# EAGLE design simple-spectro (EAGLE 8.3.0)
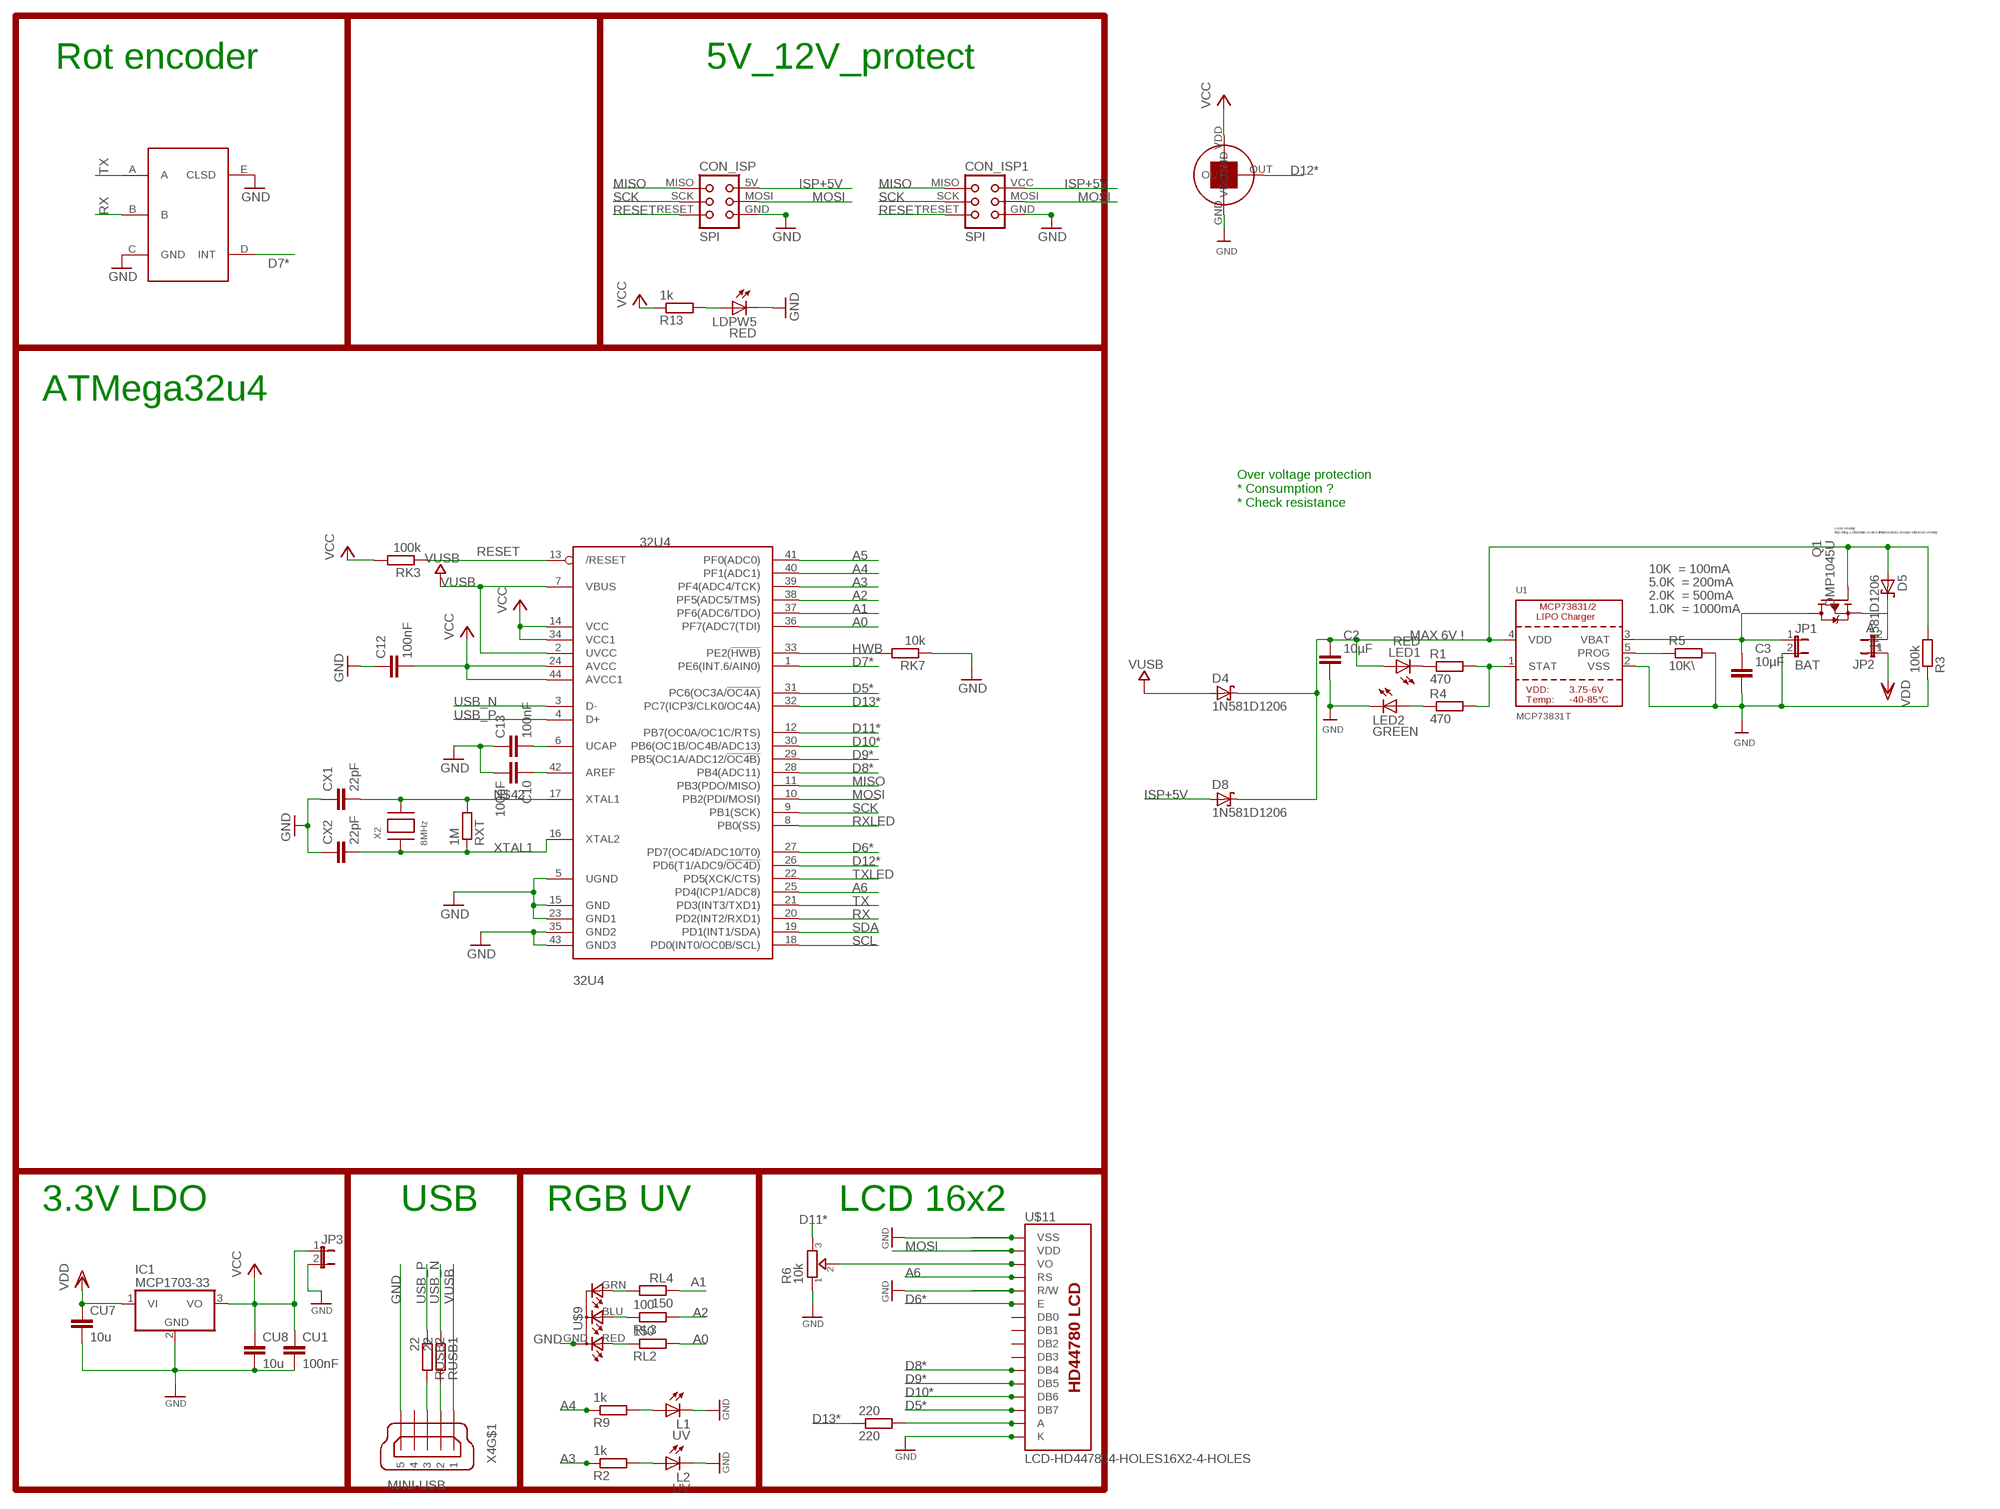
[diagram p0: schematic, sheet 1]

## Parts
32U4  32U4  ATMEGA32U4-AU  [TQFP44]
220  220  R-EU_M1206  [M1206]
C2  10µF  CAPACITOR_NPOL-1206  [C1206]
C3  10µF  CAPACITOR_NPOL-1206  [C1206]
C10  100nF  C-EUC1206  [C1206]
C12  100nF  C-EUC1206  [C1206]
C13  100nF  C-EUC1206  [C1206]
CON_ISP  SPI  TINYISPT  [TC2030-MCP-NL]
CON_ISP1  SPI  TINYISP  [TINYISP]
CU1  100nF  C-EUC1206  [C1206]
CU7  10u  C-EUC1206  [C1206]
CU8  10u  C-EUC1206  [C1206]
CX1  22pF  C-EUC1206  [C1206]
CX2  22pF  C-EUC1206  [C1206]
D4  1N581D1206  [LED-1206]
D5  1N581D1206  [LED-1206]
D8  1N581D1206  [LED-1206]
IC1  MCP1703-33  MCP1703DB  [SOT223]
JP1  BAT  JP1E  [JP1]
JP2  A  JP1E  [JP1]
JP3  JP1E  [JP1]
L1  UV  LED5MM  [LED5MM]
L2  UV  LED3MM  [LED3MM]
LDPW5  RED  LED1206  [LED-1206]
LED1  RED  LED1206  [LED-1206]
LED2  GREEN  LED1206  [LED-1206]
Q1  DMP1045U  TRANSISTOR_FET_TSM2301CX  [SOT-23]
R1  470  R-EU_M1206  [M1206]
R2  1k  R-EU_M1206  [M1206]
R3  100k  R-EU_M1206  [M1206]
R4  470  R-EU_M1206  [M1206]
R5  10K\  R-EU_M1206  [M1206]
R6  10k  TRIMMER-3362P  [TRIMMER_3362P]
R9  1k  R-EU_M1206  [M1206]
R13  1k  R-EU_M1206  [M1206]
RK3  100k  R-EU_M1206  [M1206]
RK7  10k  R-EU_M1206  [M1206]
RL2  150  R-EU_M1206  [M1206]
RL3  100  R-EU_M1206  [M1206]
RL4  150  R-EU_M1206  [M1206]
RUSB1  22  R-EU_M1206  [M1206]
RUSB2  22  R-EU_M1206  [M1206]
RXT  1M  R-EU_M1206  [M1206]
U1  MCP73831T  MCP73831/2  [SOT23-5]
U$1  EC11E  [EC11E]
U$7  TSL237  [TSL237]
U$9  RGB-COMMON-CATHODE  [LED-TRICOLOR-THROUGHHOLE]
U$11  LCD-HD447804-HOLES16X2-4-HOLES  [LCD-16X2-4HOLES]
X2  8MHz  XTALNX6035  [NX6035]
X4  MINI-USB  MINI-USB-SCHIELD-32005-201  [32005-201]

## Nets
A0: 32U4.36(PF7(ADC7(TDI)) RL2.2
A1: 32U4.37(PF6(ADC6/TDO)) RL4.1
A2: 32U4.38(PF5(ADC5/TMS)) RL3.2
A3: 32U4.39(PF4(ADC4/TCK)) R2.1
A4: 32U4.40(PF1(ADC1)) R9.1
A5: 32U4.41(PF0(ADC0))
A6: 32U4.25(PD4(ICP1/ADC8)) U$11.4(RS)
AREF: 32U4.42(AREF) C10.1
D5*: 32U4.31(PC6(OC3A/!OC4A)) U$11.14(DB7)
D6*: 32U4.27(PD7(OC4D/ADC10/T0)) U$11.6(E)
D7*: 32U4.1(PE6(INT.6/AIN0)) U$1.D(INT)
D8*: 32U4.28(PB4(ADC11)) U$11.11(DB4)
D9*: 32U4.29(PB5(OC1A/ADC12/!OC4B)) U$11.12(DB5)
D10*: 32U4.30(PB6(OC1B/OC4B/ADC13)) U$11.13(DB6)
D11*: 32U4.12(PB7(OC0A/OC1C/RTS)) R6.3
D12*: 32U4.26(PD6(T1/ADC9/!OC4D)) U$7.OUT
D13*: 32U4.32(PC7(ICP3/CLK0/OC4A)) 220.1
GND [power]: 32U4.5(UGND) 32U4.15(GND) 32U4.23(GND1) 32U4.35(GND2) 32U4.43(GND3) C2.2 C3.2 C10.2 C12.1 C13.1 CON_ISP1.GND CON_ISP.GND CU1.2 CU7.2 CU8.2 CX1.1 CX2.1 IC1.2(GND) JP1.2 JP3.2 L1.K(C) L2.K(C) LDPW5.C LED2.C R3.1 R5.2 R6.1 RK7.1 U1.2(VSS) U$1.C(GND) U$1.E(CLSD) U$7.GND U$9.GND(A2) U$11.1(VSS) U$11.5(R/W) U$11.16(K) X4.5
HWB: 32U4.33(PE2(!HWB)) RK7.2
ISP+5V: CON_ISP1.VCC CON_ISP.5V(VCC) D8.A
MISO: 32U4.11(PB3(PDO/MISO)) CON_ISP1.MISO CON_ISP.MISO
MOSI: 32U4.10(PB2(PDI/MOSI)) CON_ISP1.MOSI CON_ISP.MOSI U$11.2(VDD)
N$1: 32U4.6(UCAP) C13.2
N$2: R6.2 U$11.3(VO)
N$3: L1.A R9.2
N$4: LED1.C R1.1
N$5: R1.2 R4.2 U1.1(STAT)
N$6: R5.1 U1.5(PROG)
N$7: LED2.A R4.1
N$8: L2.A R2.2
N$9: RL4.2 U$9.GRN(CGREEN)
N$10: RL3.1 U$9.BLU(CBLUE)
N$11: 220.2 U$11.15(A)
N$12: LDPW5.A R13.2
N$13: RL2.1 U$9.RED(CRED)
N$15: C2.1 D4.C D5.A D8.C LED1.A Q1.1(G) R3.2 U1.4(VDD)
N$17 [power]: D5.C JP2.2 Q1.2(S)
N$42: 32U4.17(XTAL1) CX1.2 RXT.2 X2.P$2
RESET: 32U4.13(/RESET) CON_ISP1.RESET CON_ISP.RESET RK3.1
RX: 32U4.20(PD2(INT2/RXD1)) U$1.B
RXLED: 32U4.8(PB0(SS))
SCK: 32U4.9(PB1(SCK)) CON_ISP1.SCK CON_ISP.SCK
SCL: 32U4.18(PD0(INT0/OC0B/SCL))
SDA: 32U4.19(PD1(INT1/SDA))
TX: 32U4.21(PD3(INT3/TXD1)) U$1.A
TXLED: 32U4.22(PD5(XCK/CTS))
USB_N: 32U4.3(D-) RUSB1.1
USB_P: 32U4.4(D+) RUSB2.1
USBC_N: RUSB1.2 X4.2
USBC_P: RUSB2.2 X4.3
VBAT1: C3.1 JP1.1 Q1.3(D) U1.3(VBAT)
VCC: 32U4.14(VCC) 32U4.24(AVCC) 32U4.34(VCC1) 32U4.44(AVCC1) C12.2 CU1.1 CU8.1 IC1.3(VO) JP3.1 R13.1 RK3.2 U$7.VDD
VDD [power]: CU7.1 IC1.1(VI) JP2.1
VUSB: 32U4.2(UVCC) 32U4.7(VBUS) D4.A X4.1
XTAL1: 32U4.16(XTAL2) CX2.2 RXT.1 X2.P$1
Unconnected: U$11.7(DB0) U$11.8(DB1) U$11.9(DB2) U$11.10(DB3) X4.4 X4.M1(S:S1) X4.M2(S:S2) X4.M3(S:S3) X4.M4(S:S4)

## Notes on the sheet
- Rot encoder | 5V_12V_protect
- ATMega32u4
- Over voltage protection
  * Consumption ?
  * Check resistance
- Load sharing:
  http://blog.zakkemble.co.uk/a-lithium-battery-charger-with-load-sharing/
- 10K  = 100mA
- 5.0K  = 200mA
- 2.0K  = 500mA
- 1.0K  = 1000mA
- MAX 6V !
- 3.3V LDO | USB | RGB UV | LCD 16x2

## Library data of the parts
32U4 = adafruit:ATMEGA32U4: http://www.ladyada.net/library/eagle
220 R1-R5 R9 R13 RK3 RK7 RL2-RL4 RUSB1 RUSB2 RXT = rcl:R-EU_: RESISTOR, European symbol
C2 C3 = dp_devices:CAPACITOR_NPOL: Non-Polarized capacitor in various packages
C10 C12 C13 CU1 CU7 CU8 CX1 CX2 = resistor:C-EU: CAPACITOR, European symbol
CON_ISP = lpatiny:TINYISP: CONNECTOR
CON_ISP1 = lpatiny:TINYISP: CONNECTOR; OC_FARNELL: unknown; OC_NEWARK: unknown
D4 D5 D8 = lpatiny:1N581*: 1.0A SCHOTTKY BARRIER RECTIFIER
IC1 = linear:MCP1703: 250 mA, 16V, Low Quiescent Current LDO Regulator Source: http://ww1.microchip.com/downloads/en/DeviceDoc/22049b.pdf
JP1-JP3 = jumper:JP1E: JUMPER
L1 LDPW5 LED1 LED2 = SparkFun:LED: LEDs
L2 = led:LED: LED
Q1 = dp_devices:TRANSISTOR_FET_TSM2301CX: 20V P-Channel Enhancement Mode MOSFET
R6 = dp_devices:TRIMMER: Trimmer resistor
U1 = microbuilder:MCP73831/2: MCP73831/2 LIPO Charger VDD: 3.75 - 6V Temp -40 - 85°C Programmable Charge Rate: 15-500mA NOTE: STAT is a tri-state logic output on the MCP73831 and an open-drain output on the MCP73832. SOT23-5 with 4.2V output and tri-state logic on STAT = MCP73831T-2ACI/OT
U$1 = lpatiny:EC11E: ALPS Rotary encoder
U$7 = lpatiny:TSL237
U$9 = lpatiny:RGB-COMMON-CATHODE
U$11 = HD44780LCD:LCD-HD44780
X2 = lpatiny:XTAL: Low cost SMT crystals, no capacitors included
X4 = con-cypressindustries:MINI-USB-SCHIELD-: MINI USB-B Conector Source: www.cypressindustries.com; OC_FARNELL: unknown; OC_NEWARK: unknown

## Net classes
0 default: width 0.406 mm, clearance 0.25 mm
1 power: width 0.406 mm, drill 0.305 mm, clearance 0.25 mm
2 VIN: width 0.406 mm, clearance 0.25 mm
3 fine: width 0.406 mm, clearance 0.25 mm
4 aref: width 0.406 mm, clearance 0.25 mm

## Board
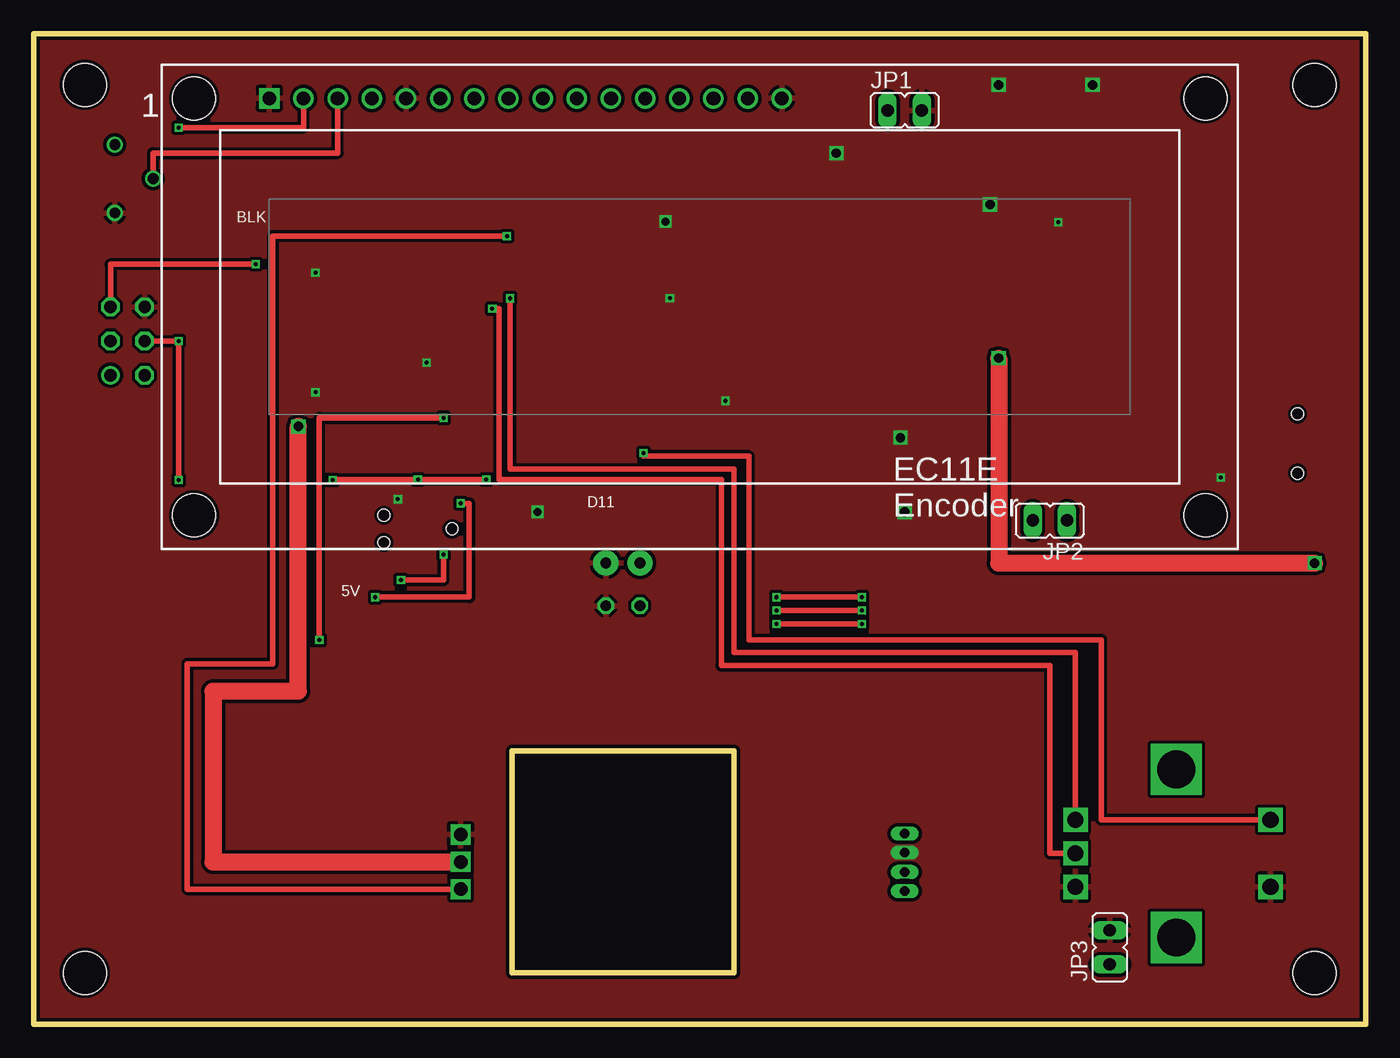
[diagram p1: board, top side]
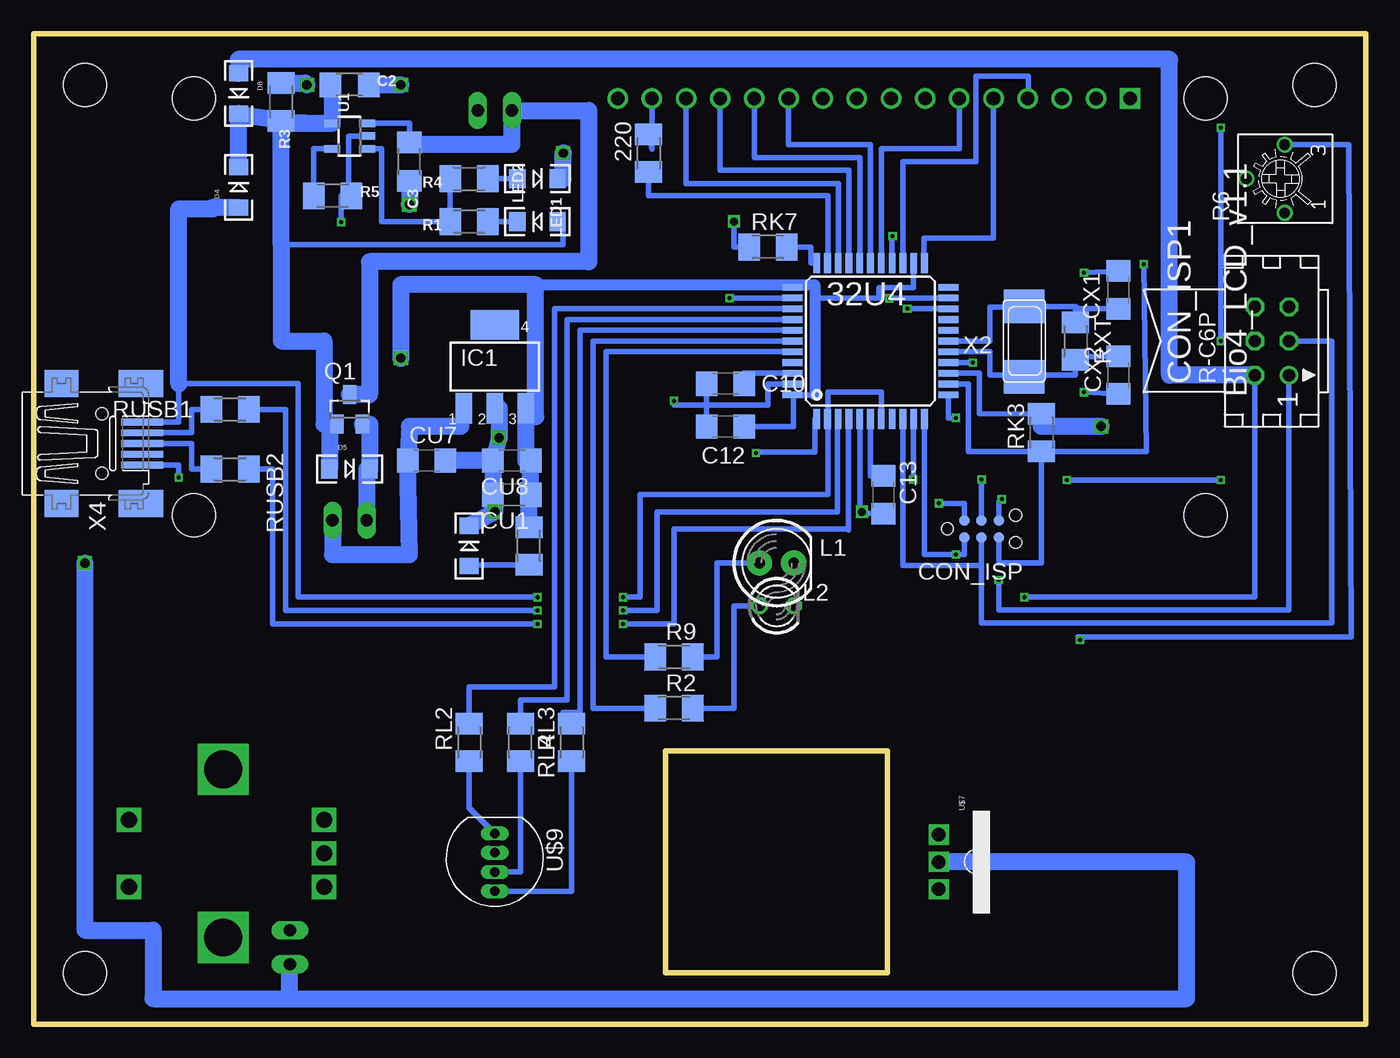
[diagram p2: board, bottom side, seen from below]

Size 99.06 x 73.66 mm. Coordinates in mm from the lower left corner, seen from the top.
Outline: 0,73.66 0,0 99.06,0 99.06,73.66 0,73.66
Outline: 35.56,20.32 52.07,20.32 52.07,3.81 35.56,3.81 35.56,20.32
Copper layers (1*2*15*16): Top 0.035mm / dielectric 0.2mm / layer 2 0.0175mm / dielectric 1.1mm / layer 15 0.0175mm / dielectric 0.2mm / Bottom 0.035mm
Design rules "SeeedStudio_DRU_no_angle_20130527": minimum track width 6mil, minimum drill 12mil, track to track 6mil, track to pad 6mil, pad to pad 6mil, via to via 6mil, smd to smd 0mil, copper to edge 10mil, drill to drill 10mil, minimum pad ring 6mil, minimum via ring 6mil, stop-mask expansion 2mil, vias tented up to drill 25mil, thermal gap 10mil
Holes 3.2 mm at 3.81,69.85 3.81,3.81 95.25,69.85 95.25,3.81

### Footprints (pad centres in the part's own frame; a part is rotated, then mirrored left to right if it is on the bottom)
TQFP44 = smd 1.5 x 0.5: 1 -5.8,4; 2 -5.8,3.2; 3 -5.8,2.4; 4 -5.8,1.6; 5 -5.8,0.8; 6 -5.8,0; 7 -5.8,-0.8; 8 -5.8,-1.6; 9 -5.8,-2.4; 10 -5.8,-3.2; 11 -5.8,-4; 23 5.8,-4; 24 5.8,-3.2; 25 5.8,-2.4; 26 5.8,-1.6; 27 5.8,-0.8; 28 5.8,0; 29 5.8,0.8; 30 5.8,1.6; 31 5.8,2.4; 32 5.8,3.2; 33 5.8,4 | smd 0.5 x 1.5: 12 -4,-5.8; 13 -3.2,-5.8; 14 -2.4,-5.8; 15 -1.6,-5.8; 16 -0.8,-5.8; 17 0,-5.8; 18 0.8,-5.8; 19 1.6,-5.8; 20 2.4,-5.8; 21 3.2,-5.8; 22 4,-5.8; 34 4,5.8; 35 3.2,5.8; 36 2.4,5.8; 37 1.6,5.8; 38 0.8,5.8; 39 0,5.8; 40 -0.8,5.8; 41 -1.6,5.8; 42 -2.4,5.8; 43 -3.2,5.8; 44 -4,5.8
M1206 = smd 1.6 x 2: 1 -1.4,0; 2 1.4,0
C1206 = smd 1.6 x 1.803: 1 -1.422,0; 2 1.422,0
C1206' = smd 1.6 x 1.8: 1 -1.4,0; 2 1.4,0
TC2030-MCP-NL = smd 0.787 x 0.787: 5V 1.27,0.635; GND 3.81,0.635; MISO 1.27,-0.635; MOSI 2.54,0.635; RESET 3.81,-0.635; SCK 2.54,-0.635 | hole 0.889: 0,0; 5.08,-1.016; 5.08,1.016
TINYISP = drill 0.914 octagon: GND 2.54,1.27; MOSI 0,1.27; RESET 2.54,-1.27; SCK 0,-1.27; VCC -2.54,1.27 | drill 0.914: MISO -2.54,-1.27
LED-1206 = smd 1.2 x 1.4: A -1.5,0; C 1.5,0
SOT223 = smd 1.219 x 2.235: 1 -2.311,-3.099; 2 0,-3.099; 3 2.311,-3.099 | smd 3.6 x 2.2: 4 0,3.099
JP1 = drill 0.914 long: 1 0,-1.27; 2 0,1.27
LED5MM = drill 0.813 pad 1.88: A -1.27,0; K 1.27,0
LED3MM = drill 0.813 octagon: A -1.27,0; K 1.27,0
SOT-23 = smd 1 x 1.4: 1 -0.95,-1.1; 2 0.95,-1.1; 3 0,1.1
TRIMMER_3362P = drill 0.8: 1 -2.54,-0.31; 2 0,2.54; 3 2.54,-0.31
SOT23-5 = smd 0.55 x 1.2: 1 -0.95,-1.3; 2 0,-1.3; 3 0.95,-1.3; 4 0.95,1.3; 5 -0.95,1.3
EC11E = drill 1.2 square: A -2.5,0; B 0,0; C 2.5,0; D -2.5,14.5; E 2.5,14.5 | drill 2.8 square: P$1 6.25,7.5; P$2 -6.25,7.5
TSL237 = drill 1 pad 1.27 square: GND -2.032,-2.54; OUT 2.032,-2.54; VDD 0,-2.54
LED-TRICOLOR-THROUGHHOLE = drill 0.7 long: BLU 2.175,0; GND -0.682,0; GRN 0.746,0; RED -2.111,0
LCD-16X2-4HOLES = drill 1.016 square: 1 -32,15.5 | drill 1.016: 2 -29.46,15.5; 3 -26.92,15.5; 4 -24.38,15.5; 5 -21.84,15.5; 6 -19.3,15.5; 7 -16.76,15.5; 8 -14.22,15.5; 9 -11.68,15.5; 10 -9.14,15.5; 11 -6.6,15.5; 12 -4.06,15.5; 13 -1.52,15.5; 14 1.02,15.5; 15 3.56,15.5; 16 6.1,15.5 | hole 3.2: -37.6,15.5; -37.6,-15.5; 37.6,-15.5; 37.6,15.5
NX6035 = smd 2.5 x 3: P$1 2.665,0; P$2 -2.565,0
32005-201 = smd 3.1 x 0.5: 1 3,1.6; 2 3,0.8; 3 3,0; 4 3,-0.8; 5 3,-1.6 | smd 2.5 x 2: M1 -3,-4.45; M2 -3,4.45 | smd 3.3 x 2: M3 2.9,4.45; M4 2.9,-4.45 | hole 0.9: 0,2.2; 0,-2.2

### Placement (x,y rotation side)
32U4  36.83,50.8 90 bottom
220  53.34,64.77 90 bottom
C2  75.56,69.85 0 bottom
C3  71.12,64.14 270 bottom
C10  100nF  [C1206']  47.62,47.62 180 bottom
C12  100nF  [C1206']  47.62,44.45 0 bottom
C13  100nF  [C1206']  35.88,39.37 90 bottom
CON_ISP  31.11,36.83 0 bottom
CON_ISP1  6.99,50.8 90 bottom
CU1  100nF  [C1206']  63.5,39.37 180 bottom
CU7  10u  [C1206']  69.85,41.91 0 bottom
CU8  10u  [C1206']  63.5,41.91 180 bottom
CX1  22pF  [C1206']  18.41,54.61 270 bottom
CX2  22pF  [C1206']  18.41,48.26 90 bottom
D4  83.82,62.23 90 bottom
D5  75.56,41.27 0 bottom
D8  83.82,69.22 270 bottom
IC1  64.77,48.9 0 bottom
JP1  64.77,67.94 270 top
JP2  75.56,37.47 90 top
JP3  80.01,5.71 0 top
L1  43.81,34.29 0 bottom
L2  43.81,31.11 0 bottom
LDPW5  66.67,35.56 90 bottom
LED1  61.59,59.69 180 bottom
LED2  61.59,62.87 0 bottom
Q1  75.56,45.72 0 bottom
R1  66.67,59.69 180 bottom
R2  51.44,23.5 0 bottom
R3  80.64,68.58 270 bottom
R4  66.67,62.87 180 bottom
R5  76.83,61.59 0 bottom
R6  6.35,62.87 90 bottom
R9  51.44,27.3 0 bottom
R13  62.23,35.56 270 bottom
RK3  24.13,43.99 90 bottom
RK7  44.45,57.78 0 bottom
RL2  66.67,20.95 90 bottom
RL3  59.05,20.95 90 bottom
RL4  62.87,20.95 270 bottom
RUSB1  84.45,45.72 180 bottom
RUSB2  84.45,41.27 180 bottom
RXT  21.59,50.8 90 bottom
U1  75.56,66.04 90 bottom
U$1  77.47,12.7 270 top
U$7  29.21,12.06 270 bottom
U$9  64.77,12.06 270 bottom
U$11  49.53,53.34 0 top
X2  25.4,50.8 270 bottom
X4  93.98,43.18 0 bottom

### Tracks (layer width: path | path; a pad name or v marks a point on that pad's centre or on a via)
A0
  Bottom 0.406: 32U4.36 60.33,53.2 60.33,25.07 66.67,25.07 RL2.2
A1
  Bottom 0.406: 32U4.37 59.41,52.4 59.41,24.13 62.87,24.13 RL4.1
A2
  Bottom 0.406: 32U4.38 58.42,51.6 58.42,23.19 59.69,23.19 RL3.2
A3
  Bottom 0.406: 32U4.39 57.48,50.8 57.48,23.5 R2.1
A4
  Bottom 0.406: 42.63,50.04 32U4.40 56.52,50 56.52,27.3 R9.1
A6
  Bottom 0.406: U$11.4 25.08,68.84 25.08,70.48 29,70.48 29,64.14 34.43,64.14 32U4.25
AREF
  Bottom 0.406: 32U4.42 46.23,48.4 C10.1
D5*
  Bottom 0.406: 39.24,56.6 32U4.31 39.23,62.5 50.55,62.5 U$11.14
D6*
  Bottom 0.406: 32U4.27 36.03,65.09 30.23,65.09 U$11.6
D7*  (via drill 0.3)
  Top 0.406: U$1.D 79.38,15.2 79.38,28.57 53.17,28.57 53.17,42.24 45.34,42.24 v45.34,42.48
  Bottom 0.406: 32U4.1 40.96,45 40.96,42.55 45.34,42.55 v45.34,42.48 | 91.97,14.93 U$1.D
D8*
  Bottom 0.406: 32U4.28 36.83,65.41 42.93,65.41 U$11.11
D9*
  Bottom 0.406: 32U4.29 37.63,64.45 45.47,64.45 U$11.12
D10*
  Bottom 0.406: 32U4.30 38.43,63.5 48.01,63.5 U$11.13
D11*  (via drill 0.3)
  Top 0.406: v21.25,28.57 21.25,45.09 v30.48,45.09
  Bottom 0.406: R6.3 1.27,65.41 1.1,28.8 21.42,28.8 v21.25,28.57 | v30.48,45.09 31.03,45.09 32U4.12
D12*  (via drill 0.3)
  Top 0.406: v35.19,58.61 17.78,58.61 17.78,26.8 11.43,26.8 11.43,10.03 U$7.OUT
  Bottom 0.406: 32U4.26 35.24,58.51 35.19,58.51 v35.19,58.61
D13*
  Bottom 0.406: 32U4.32 40.01,56.6 40.01,61.59 53.34,61.59 220.1
GND  (via drill 0.3, 0.6, 0.7)
  Bottom 0.406: 49.02,47.6 C10.2 49.02,46.04 | 49.02,46.04 C12.1 | 32U4.43 44.45,47.6 44.45,46.04 49.02,46.04 | v51.44,46.35 51.44,46.04 49.02,46.04 | C13.1 37.47,37.97 | 32U4.5 37.63,37.97 37.47,37.97 | U$11.5 27.69,58.45 32.85,58.45 32.85,56.6 32U4.23 | 64.77,41.91 CU8.2 | CU1.2 64.77,39.37 | X4.5 88.27,41.58 v88.27,40.64 | 32U4.35 v47.3,54 | CX1.1 v20.95,55.88 | 32U4.15 v29.22,49.2 | v29.22,49.2 | CON_ISP.GND 27.3,38.81 v27.08,39.04 | RK7.1 46.99,57.78 v46.99,59.69 | 37.47,37.97 v37.47,38.1 | CX2.1 v20.95,46.99 | 75.65,61.59 R5.2 | 75.65,61.59 76.2,61.59 v76.2,59.64 | U1.2 75.65,66.04 75.65,61.59
  Bottom 1.27: LED2.C 59.69,62.87 v59.69,64.77 | C3.2 v71.12,60.96 | 64.45,45.16 IC1.2 64.45,45.8 v64.45,43.62 CU8.2 | CU8.2 CU7.2 | CU8.2 CU1.2 | LDPW5.C v64.77,38.1 64.77,39.37 | C2.2 v71.75,69.85 | R3.1 78.87,69.98 v78.74,69.85
  pour Top: 0,73.66 0,0 99.06,0 99.06,73.66
HWB
  Bottom 0.406: 32U4.33 41.27,56.6 41.27,57.78 RK7.2
ISP+5V  (via drill 0.3)
  Top 0.406: v31.75,38.73 32.38,38.73 32.38,31.75 v25.4,31.75
  Bottom 0.406: CON_ISP.5V 29.84,38.73 v31.75,38.73 | v25.4,31.75 8.26,31.75 CON_ISP1.VCC
  Bottom 1.27: CON_ISP1.VCC 14.61,48.26 14.61,71.75 83.82,71.75 D8.A
MISO  (via drill 0.3)
  Top 0.406: v27.3,33.02 30.48,33.02 v30.48,34.92
  Bottom 0.406: CON_ISP.MISO 29.84,34.92 v30.48,34.92 32.83,34.92 32U4.11 | CON_ISP1.MISO 5.71,30.79 27.3,30.79 v27.3,33.02
MOSI  (via drill 0.3)
  Top 0.406: v33.66,40.5 v28.57,40.5 22.23,40.5 v22.23,40.47 | CON_ISP1.MOSI v10.79,50.8 v10.79,40.47 | v10.79,66.67 20.07,66.67 U$11.2
  Bottom 0.406: CON_ISP.MOSI v28.57,40.5 | v10.79,50.8 v10.79,66.67 | v22.23,40.47 v10.79,40.47 | 32U4.10 33.63,40.52 v33.66,40.5
N$1
  Bottom 0.406: C13.2 36.83,40.77 32U4.6
N$2
  Top 0.406: R6.2 8.89,64.77 22.61,64.77 U$11.3
  Bottom 0.406: U$11.3
N$3
  Bottom 0.406: R9.2 48.26,27.3 48.26,34.29 L1.A
N$4
  Bottom 0.406: LED1.C R1.1
N$5
  Bottom 0.406: R4.2 R1.2 73.19,59.69 73.19,65.09 U1.1
N$6
  Bottom 0.406: U1.5 78.23,65.09 R5.1
N$7
  Bottom 0.406: R4.1 LED2.A
N$8
  Bottom 0.406: R2.2 46.99,23.5 46.99,31.11 L2.A
N$9
  Bottom 0.406: U$9.GRN 62.87,11.32 RL4.2
N$10
  Bottom 0.406: RL3.1 59.05,9.89 U$9.BLU
N$11
  Bottom 0.406: U$11.15 53.09,65.08 220.2
N$12
  Bottom 0.406: R13.2 66.67,34.16 LDPW5.A
N$13
  Bottom 0.406: RL2.1 66.67,16.08 U$9.RED
N$15
  Bottom 0.406: C2.1 76.86,69.85 | 77.06,44.62 Q1.1 | LED1.A 59.69,59.69 59.69,57.96 80.64,57.96
  Bottom 1.27: D4.C D8.C 83.82,67.63 R3.2 80.64,66.99 78.76,66.99 | 77.06,44.62 D5.A | 77.06,44.62 77.47,44.62 77.47,50.8 80.64,50.8 80.64,57.96 80.64,66.97 78.76,66.99 | 76.86,69.85 U1.4 78.76,66.99
N$17
  Bottom 1.27: Q1.2 74.06,44.62 D5.C 74.3,41.27 JP2.2
N$42
  Bottom 0.406: 32U4.17 27.94,50.8 27.94,53.34 25.4,53.34 X2.P$2 21.59,53.37 | 21.59,53.37 RXT.2 | CX1.2 21.43,53.21 21.59,53.37
RESET  (via drill 0.3)
  Top 0.406: v16.51,56.52 5.71,56.52 CON_ISP1.RESET
  Bottom 0.406: 32U4.13 29.54,47.6 29.54,42.57 RK3.1 | CON_ISP.RESET 27.3,34.29 24.13,34.29 RK3.1 | RK3.1 16.34,42.57 v16.51,56.52
RX  (via drill 0.3)
  Top 0.406: v34.1,53.21 34.62,53.21 34.62,40.5 51.13,40.5 51.13,26.67 75.56,26.67 75.56,12.7 U$1.B
  Bottom 0.406: 32U4.20 v34.1,53.2 v34.1,53.21
SCK
  Bottom 0.406: CON_ISP.SCK 28.57,34.12 | 28.57,34.12 34.43,34.12 32U4.9 | CON_ISP1.SCK 2.54,50.8 2.54,29.84 28.57,29.84 28.57,34.12
TX  (via drill 0.3)
  Top 0.406: v35.42,53.98 35.42,41.27 52.07,41.27 52.07,27.64 77.47,27.64 U$1.A
  Bottom 0.406: 32U4.21 v35.42,53.98
USB_N  (via drill 0.3)
  Top 0.406: v55.24,30.76 v61.58,30.76
  Bottom 0.406: 32U4.3 39.29,45 39.29,38.1 52.7,38.1 52.7,30.76 v55.24,30.76 | v61.58,30.76 80.33,30.76 80.33,45.72 RUSB1.1
USB_P  (via drill 0.3)
  Top 0.406: v55.24,29.77 v61.58,29.77
  Bottom 0.406: 32U4.4 38.47,45 38.47,36.83 | v61.58,29.77 81.28,29.77 81.28,41.27 RUSB2.1 | v55.24,29.77 51.44,29.77 51.44,36.83 38.47,36.83 | 38.47,36.83 38.47,36.75
USBC_N
  Bottom 0.406: X4.2 87.3,43.98 87.3,45.72 RUSB1.2
USBC_P
  Bottom 0.406: X4.3 87.3,43.18 87.3,41.27 RUSB2.2
VBAT1
  Bottom 0.406: U1.3 71.12,66.99 71.12,65.41
  Bottom 1.27: C3.1 71.12,65.41 63.5,65.41 JP1.1 57.78,67.94 57.78,56.69 74.08,56.69 74.08,46.81 75.56,46.81 Q1.3
VCC  (via drill 0.7)
  Top 1.27: v71.75,49.53 71.75,34.29 v95.25,34.29 | v19.68,44.45 19.68,24.77 13.34,24.77 13.34,12.06 U$7.VDD
  Bottom 0.406: C12.2 42.55,44.45 42.55,46.8 32U4.44 40.98,46.8 40.8,53.98 | 32U4.14 28.74,48.4 28.74,45.4 RK3.2 | 40.8,53.98 40.8,54.8 32U4.34 | 32U4.24 33.66,56.6 33.66,54.77 36.22,54.77 36.22,53.98 40.8,53.98
  Bottom 0.813: IC1.3 62.23,45.16 | 61.72,54.98 40.98,54.98 40.98,46.8
  Bottom 1.27: R13.1 62.23,39.37 CU1.1 CU8.1 62.46,41.91 IC1.3 61.72,45.16 61.72,54.98 71.75,54.98 v71.75,49.53 | v95.25,34.29 95.25,6.99 90.17,6.99 90.17,1.91 80.01,1.91 | U$7.VDD 13.34,12.06 13.34,1.91 80.01,1.91 | v19.68,44.45 24.13,44.45 RK3.2 | 80.01,1.91 JP3.1
VDD
  Bottom 0.406: 67.31,44.45 IC1.1 67.31,45.16
  Bottom 1.27: JP2.1 76.83,34.92 71.12,34.92 CU7.1 71.12,44.45 67.31,44.45
VUSB  (via drill 0.3)
  Top 0.406: v55.24,31.75 v61.58,31.75
  Bottom 0.406: 40.01,45 40.01,46.99 36.03,46.99 32U4.7 | 32U4.2 40.01,45 | 40.01,45 40.01,39.37 53.98,39.37 53.98,31.75 v55.24,31.75 | v61.58,31.75 79.38,31.75 79.38,47.62 88.27,47.62 88.27,44.78 X4.1 | 85.72,60.73 85.72,60.63
  Bottom 1.27: 88.27,47.62 88.27,60.63 85.72,60.63 | D4.A 85.72,60.73
XTAL1
  Bottom 0.406: 25.4,48.26 21.59,48.26 RXT.1 21.59,49.66 CX2.2 | 25.4,48.26 X2.P$1 | 25.4,48.26 27.94,48.26 27.94,50 32U4.16

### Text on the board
tNames: 1 | BLK | D11 | EC11E / Encoder | 5V
bNames: Bio4_LCD_v1.1
tValues: Simple spectrophotometer V 1.2.0
bValues: Simple spectrophotometer V 1.2.0

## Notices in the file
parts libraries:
lpatiny: ©2009 ROFA.cz - modified and updated by Robert Darlington ‹rdarlington@gmail.com›
microbuilder: This work is placed in the public domain, and may be freely used for commercial and non-commercial work with the following conditions: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
